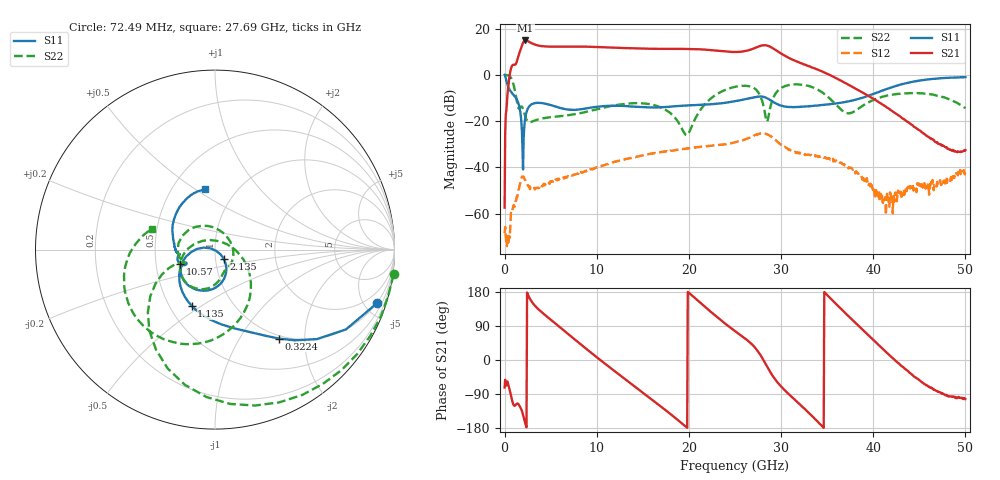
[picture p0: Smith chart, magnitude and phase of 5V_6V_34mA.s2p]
! MARKI MICROWAVE INC.
! Date:  1/07/2020
! Model Number:  APM-6849CH
! Description:  2-port Small Signal S-parameter data for APM-6849CH
! Frequency Range:  10 MHz to 50 GHz
! Port Configuration:  PORT 1: Input
!  PORT 2: Output
! Bias Condition: Vc = +5V, Vb = +6V
! APM-6849CH s2p files are only valid for small signal conditions (below -5 dBm input power)
!S2P File: Measurements: Mag<S11> Ang<S11>, Mag<S21> Ang<S21>, Mag<S12> Ang<S12>, Mag<S22> Ang<S22>!row 1
# Hz S  dB  R 50
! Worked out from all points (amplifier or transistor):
!   801 points, 10 MHz to 50 GHz, reference 50 ohm
!   highest |S21| = 14.9 dB at 2.26 GHz (marker M1)
!   |S21| within 3 dB of that: 1.823 GHz to 11.14 GHz (9.317 GHz wide, 144 % of centre)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
!   unconditionally stable (mu >= 1): 125.6 MHz to end of sweep
!   at 8.321 GHz: K = 14.41, MAG = 12.5 dB, |S12| = -41.9 dB
!   at 25 GHz: K = 3.01, MAG = 11.8 dB, |S12| = -29.2 dB
!   at 50 GHz: K = 503.98, MAG = -25.4 dB, |S12| = -41.8 dB
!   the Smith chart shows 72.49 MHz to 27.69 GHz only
!   S11 on the Smith chart (normalised r, x): 72.49 MHz: 0.98, -6.03; 322.4 MHz: 0.95, -1.50; 1.135 GHz: 0.64, -0.46; 2.135 GHz: 1.10, -0.11; 10.57 GHz: 0.67, -0.11; 27.69 GHz: 0.72, +0.55
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1e7  -0.02 -2.8  -57.34 -72.7  -68.35 136.0  0.04 -1.1
7.24875e7  -0.45 -18.4  -25.41 -52.2  -65.70 -26.5  0.04 -7.9
3.224375e8  -4.30 -54.4  -8.14 -56.8  -68.95 29.0  -0.15 -36.4
1.134775e9  -9.40 -112.5  4.34 -120.6  -55.41 -50.8  -7.03 -144.1
1.822138e9  -19.98 177.8  11.85 -130.4  -44.90 -99.3  -13.62 -178.1
2.134575e9  -22.91 -46.3  14.62 -156.7  -44.71 -143.9  -16.41 118.5
2.25955e9  -18.43 -58.2  14.86 -168.0  -45.48 -153.4  -18.04 95.1
2.946912e9  -12.70 -100.6  13.66 154.1  -48.54 -168.5  -20.20 10.8
4.321638e9  -12.36 -138.9  12.29 120.2  -47.53 -178.2  -18.68 -38.6
8.383325e9  -14.78 -152.8  12.21 39.0  -42.22 136.9  -16.42 -75.5
1.057039e10  -13.55 -158.0  11.94 -3.5  -39.19 109.4  -14.35 -89.1
1.381974e10  -13.68 -170.5  11.47 -64.2  -35.82 67.2  -12.29 -120.0
1.669416e10  -14.06 -172.5  11.24 -117.6  -33.45 25.4  -13.64 -158.5
2.038092e10  -13.10 179.2  11.14 169.4  -31.52 -32.4  -21.60 15.3
2.269296e10  -12.57 168.6  10.59 120.7  -30.44 -73.8  -9.24 -57.0
2.5005e10  -11.38 151.1  9.88 76.3  -29.16 -117.7  -5.17 -107.3
2.769196e10  -9.34 99.4  12.42 15.9  -25.45 163.8  -8.67 161.7
2.944161e10  -12.37 51.0  10.67 -53.8  -28.15 89.9  -7.88 -77.9
3.337832e10  -13.44 -0.4  3.16 -148.1  -34.59 11.3  -5.31 -178.5
3.644021e10  -12.07 -23.0  -2.40 136.5  -38.08 -60.6  -14.78 159.9
4.168916e10  -5.80 -39.2  -14.58 14.3  -55.34 77.2  -8.83 -176.3
5e10  -0.97 -97.8  -32.51 -102.9  -41.83 -73.8  -14.43 63.6
